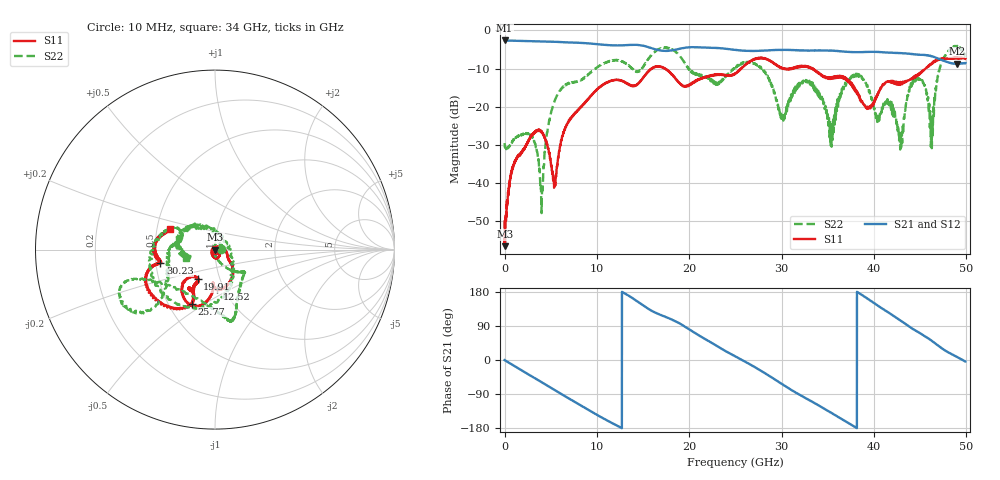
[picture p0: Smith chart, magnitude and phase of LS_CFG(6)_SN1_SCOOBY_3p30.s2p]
!Keysight Technologies,N5245B,MY58422026,A.13.80.08
!Date: Thursday, March 19, 2020 23:28:31
!Correction: S11(Full 2 Port(1,2))
!S21(Full 2 Port(1,2))
!S12(Full 2 Port(1,2))
!S22(Full 2 Port(1,2))
!S2P File: Measurements: S11, S21, S12, S22:
# Hz S DB R 50.0
!freq dBS11 angS11 dBS21 angS21 dBS12 angS12 dBS22 angS22
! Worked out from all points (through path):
!   4991 points, 10 MHz to 49.91 GHz, reference 50 ohm
!   highest |S21| = -2.64 dB at 10 MHz (marker M1); lowest = -8.7 dB at 49.01 GHz (marker M2)
!   group delay of S21, straight-line fit = 39.9 ps
!   lowest |S11| = -56.5 dB at 50 MHz (marker M3), VSWR 1.00, Z = 50.1 + j0.0414 ohm
!   |S11| at or under -10 dB: start of sweep to 15.94 GHz; 17.42 GHz to 25.59 GHz (8.172 GHz wide, 38 % of centre); 33.42 GHz to 45.62 GHz (12.2 GHz wide, 30.9 % of centre)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
!   |S22| runs from -47.8 to -4.0 dB; largest |S21 - S12| = 0.0068
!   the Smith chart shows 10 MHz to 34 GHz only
!   S11 on the Smith chart (normalised r, x): 10 MHz: 1.00, -0.01; 12.52 GHz: 0.93, -0.43; 19.91 GHz: 0.78, -0.27; 25.77 GHz: 0.66, -0.44; 30.23 GHz: 0.53, -0.09; 34 GHz: 0.58, +0.14
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1e7  -50.02 -86.4  -2.64 -0.3  -2.63 -0.3  -29.50 3.5
5e7  -56.46 16.0  -2.65 -0.8  -2.64 -0.8  -30.48 -4.5
2.88e9  -27.64 -54.7  -2.81 -42.1  -2.81 -42.1  -27.46 60.2
4.02e9  -26.47 -90.3  -2.86 -58.7  -2.86 -58.6  -47.82 174.3
5.4e9  -40.51 125.2  -2.97 -79.1  -2.97 -79.1  -18.65 -58.3
8.33e9  -20.03 -37.4  -3.28 -121.0  -3.28 -120.9  -12.89 -48.2
1.252e10  -13.10 -87.1  -3.93 -177.5  -3.93 -177.5  -7.92 -79.3
1.665e10  -9.46 -113.4  -5.14 121.5  -5.13 121.5  -4.99 -158.2
1.991e10  -14.43 -120.5  -4.44 82.2  -4.43 82.3  -9.74 -147.3
2.496e10  -11.41 -117.1  -5.08 9.8  -5.07 9.9  -9.85 170.1
2.577e10  -9.70 -112.9  -5.30 -0.8  -5.29 -0.6  -8.44 -165.1
3.023e10  -10.10 -166.3  -5.10 -66.2  -5.10 -66.0  -22.75 45.3
3.328e10  -9.87 166.2  -5.28 -109.9  -5.28 -109.6  -13.87 -176.7
3.4e10  -11.07 155.7  -5.29 -119.7  -5.27 -119.3  -15.72 -160.4
3.541e10  -12.57 135.1  -5.28 -140.0  -5.24 -139.6  -30.38 174.5
3.781e10  -15.17 102.3  -5.70 -174.7  -5.65 -174.9  -11.63 172.9
4.16e10  -13.28 43.1  -5.83 124.9  -5.84 124.7  -18.78 76.5
4.294e10  -14.08 32.2  -5.96 103.4  -5.99 103.2  -30.21 34.6
4.493e10  -11.17 -8.7  -6.35 71.8  -6.37 71.8  -12.72 19.9
4.627e10  -8.54 -16.4  -6.75 50.4  -6.77 50.4  -30.83 -32.2
4.901e10  -7.06 -46.8  -8.75 7.8  -8.76 7.8  -4.04 -44.9
4.991e10  -7.44 -43.9  -8.54 -4.0  -8.56 -4.1  -6.72 -24.7
